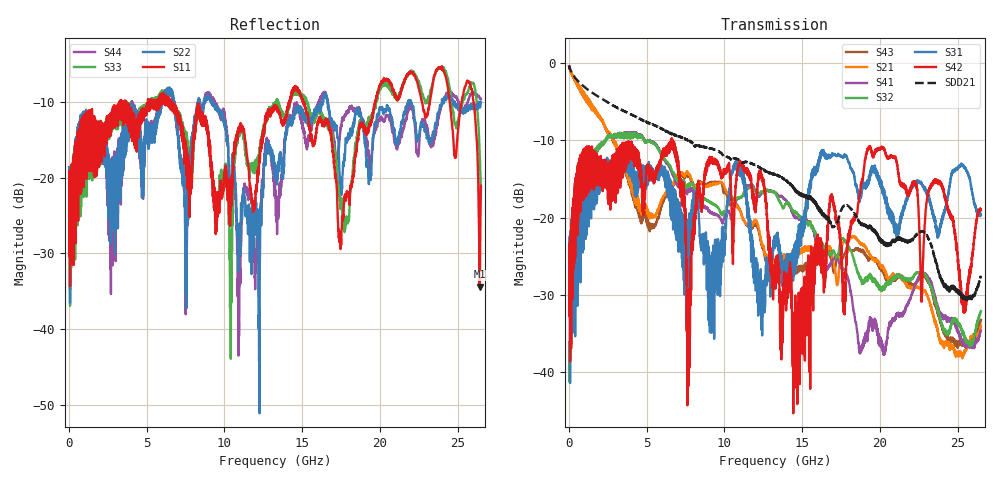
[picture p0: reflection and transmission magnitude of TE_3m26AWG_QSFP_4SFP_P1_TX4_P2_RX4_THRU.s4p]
!Agilent Technologies,N5222A,MY51421691,A.10.00.00
!Agilent N5222A: A.10.00.00
!Date: Friday, January 30, 2015 12:33:22
!Correction: S11(Full 4 Port(1,2,3,4))
!S12(Full 4 Port(1,2,3,4))
!S13(Full 4 Port(1,2,3,4))
!S14(Full 4 Port(1,2,3,4))
!S21(Full 4 Port(1,2,3,4))
!S22(Full 4 Port(1,2,3,4))
!S23(Full 4 Port(1,2,3,4))
!S24(Full 4 Port(1,2,3,4))
!S31(Full 4 Port(1,2,3,4))
!S32(Full 4 Port(1,2,3,4))
!S33(Full 4 Port(1,2,3,4))
!S34(Full 4 Port(1,2,3,4))
!S41(Full 4 Port(1,2,3,4))
!S42(Full 4 Port(1,2,3,4))
!S43(Full 4 Port(1,2,3,4))
!S44(Full 4 Port(1,2,3,4))
!S4P File: Measurements: <S11,S12,S13,S14>,
!<S21,S22,S23,S24>,
!<S31,S32,S33,S34>,
!<S41,S42,S43,S44>:
# Hz S  dB  R 50.0
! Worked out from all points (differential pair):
!   2650 points, 10 MHz to 26.5 GHz, reference 50 ohm
!   strongest paths, dB at 10 MHz, 6.63 GHz, 13.26 GHz, 19.88 GHz, 26.5 GHz:
!     S42: -25.0, -10.9, -25.5, -11.1, -19.1
!     S31: -24.8, -19.1, -23.2, -14.9, -19.7
!     S32: -39.5, -13.9, -16.8, -29.0, -32.1
!     S41: -39.5, -14.1, -16.8, -35.3, -34.6
!     S21: -0.4, -16.0, -25.4, -25.7, -34.0
!     S43: -0.4, -16.2, -26.9, -26.1, -33.3
!   taken as a pair (ports 1,3 in; 2,4 out), SDD21 dB: -0.3, -9.2, -14.4, -22.6, -27.5
!   lowest |S11| = -34.4 dB at 26.43 GHz (marker M1), VSWR 1.04, Z = 50.5 - j1.83 ohm
!   |S11| at or under -10 dB: start of sweep to 3.279 GHz; 6.607 GHz to 14.16 GHz (7.55 GHz wide, 72.7 % of centre); 15.1 GHz to 19.69 GHz (4.586 GHz wide, 26.4 % of centre)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
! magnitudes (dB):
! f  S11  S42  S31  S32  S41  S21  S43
! 10 MHz  -19.2  -25.0  -24.8  -39.5  -39.5  -0.4  -0.4
! 4.19 GHz  -11.6  -10.9  -14.1  -9.5  -9.4  -16.6  -17.1
! 7.7 GHz  -17.8  -35.6  -29.7  -15.6  -16.3  -14.5  -14.7
! 10.95 GHz  -13.9  -13.0  -13.8  -17.4  -17.5  -18.9  -18.8
! 14.56 GHz  -8.2  -30.1  -23.3  -19.3  -19.9  -24.3  -26.3
! 26.43 GHz  -34.4  -19.1  -19.4  -32.5  -35.1  -34.6  -33.6
! 26.5 GHz  -21.1  -19.1  -19.7  -32.1  -34.6  -34.0  -33.3
